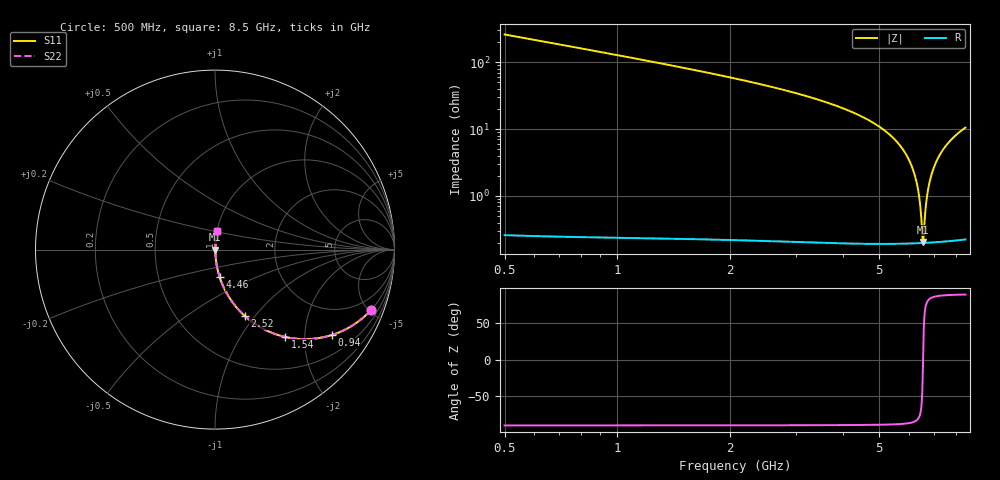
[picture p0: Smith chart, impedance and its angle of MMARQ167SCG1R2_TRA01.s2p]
! MMARQ167SCG1R2_TRA01  S-PARAMETER MODEL  ( General Type )
! Model Generated by TAIYO YUDEN Corporation (http://www.ty-top.com)
! Version 1.0
! TAIYO YUDEN Control No. 150305
! Copyright(c) 2015 TAIYO YUDEN CO.,LTD. All Rights Reserved.
! Product Description (link to TY-COMPAS)
! https://ds.yuden.co.jp/TYCOMPAS/or/detail?pn=MMARQ167SCG1R2BTRA01&u=M
! Products Name : Multilayer Ceramic Capacitors
! Characteristics :
!  Capacitance : 1.2 pF , Rated Voltage : 250V , TCC : CG / C0G
!  Case Size : 1.6 x 0.8 / 0.063 x 0.031 [mm/inch] , Thickness : 0.7 / 0.028 [mm/inch]
!  (Conditions: Temperature = 25 degC , DC Bias Current/Voltage = 0A / 0V)
! External Node Assignments :
!  1  o---| |---o  2
! GND o---------o GND
! Frequency Range : 500MHz  -  8.5GHz  [ 401 STEP ]
# MHz S RI R 50
! Freq[MHz].  S11 Real  S11 Imag  S21 Real  S21 Imag  S12 Real  S12 Imag  S22 Real  S22 Imag
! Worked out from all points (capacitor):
!   401 points, 500 MHz to 8.5 GHz, reference 50 ohm
!   read as one part in series: C = 1.22 pF near 540 MHz
!   lowest |Z| = 205 mohm at 6.56 GHz (marker M1)
!   series resonance near 6.552 GHz, so ESL is about 480 pH
!   S11 on the Smith chart (normalised r, x): 500 MHz: 1.01, -5.19; 940 MHz: 1.00, -2.72; 1.54 GHz: 1.00, -1.60; 2.52 GHz: 1.00, -0.88; 4.46 GHz: 1.00, -0.31; 8.5 GHz: 1.00, +0.21
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500  0.8706 -0.3351  0.1294 0.3351  0.1294 0.3351  0.8706 -0.3351
940  0.6492 -0.4763  0.3508 0.4763  0.3508 0.4763  0.6492 -0.4763
1540  0.3915 -0.4867  0.6085 0.4867  0.6085 0.4867  0.3915 -0.4867
1840  0.3003 -0.4567  0.6997 0.4567  0.6997 0.4567  0.3003 -0.4567
2520  0.1646 -0.3684  0.8354 0.3684  0.8354 0.3684  0.1646 -0.3684
3180  0.0914 -0.285  0.9086 0.285  0.9086 0.285  0.0914 -0.285
4460  0.026 -0.153  0.974 0.153  0.974 0.153  0.026 -0.153
4500  0.0248 -0.1495  0.9752 0.1495  0.9752 0.1495  0.0248 -0.1495
5300  0.00911 -0.0844  0.9909 0.0844  0.9909 0.0844  0.00911 -0.0844
5840  0.00404 -0.0458  0.996 0.0458  0.996 0.0458  0.00404 -0.0458
6100  0.00276 -0.0284  0.9972 0.0284  0.9972 0.0284  0.00276 -0.0284
6300  0.00221 -0.0156  0.9978 0.0156  0.9978 0.0156  0.00221 -0.0156
6400  0.00206 -0.00934  0.9979 0.00934  0.9979 0.00934  0.00206 -0.00934
6460  0.00201 -0.00562  0.998 0.00562  0.998 0.00562  0.00201 -0.00562
6520  0.00198 -0.00194  0.998 0.00194  0.998 0.00194  0.00198 -0.00194
6560  0.00198 0.000492  0.998 -0.000492  0.998 -0.000492  0.00198 0.000492
6680  0.00205 0.00771  0.9979 -0.00771  0.9979 -0.00771  0.00205 0.00771
6780  0.00219 0.0136  0.9978 -0.0136  0.9978 -0.0136  0.00219 0.0136
6940  0.00254 0.0229  0.9975 -0.0229  0.9975 -0.0229  0.00254 0.0229
7180  0.00338 0.0364  0.9966 -0.0364  0.9966 -0.0364  0.00338 0.0364
7720  0.0064 0.0653  0.9936 -0.0653  0.9936 -0.0653  0.0064 0.0653
8500  0.0131 0.1036  0.9869 -0.1036  0.9869 -0.1036  0.0131 0.1036
